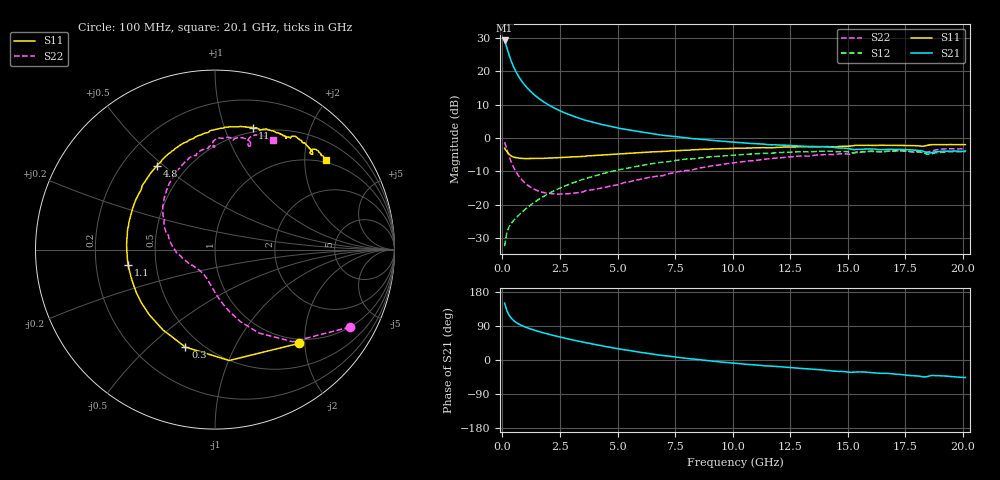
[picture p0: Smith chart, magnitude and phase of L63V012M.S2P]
!  Infineon Technologies AG
! BFR380L3 , PF131585-7, No.6, Th 09.10.01, soldered on pcb-board, measured with PP GSG850
!  Vce=3.0 V,  Ic=12.5 mA
! Common Emitter S-Parameters:  15. November 2001
#  GHz  S  MA  R  50
! f  S11  S21  S12  S22
! GHz  Mag  Ang  Mag  Ang  Mag  Ang  Mag  Ang
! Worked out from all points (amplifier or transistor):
!   201 points, 100 MHz to 20.1 GHz, reference 50 ohm
!   highest |S21| = 29.2 dB at 100 MHz (marker M1)
!   |S21| within 3 dB of that: start of sweep to 232.5 MHz
!   unconditionally stable (mu >= 1): 1.713 GHz to 4.436 GHz
!   at 3.4 GHz: K = 1.02, MAG = 8.2 dB, |S12| = -12.6 dB
!   at 10.1 GHz: K = 0.95, MSG = 1.9 dB, |S12| = -5.1 dB
!   at 20.1 GHz: K = 0.99, MSG = 0.1 dB, |S12| = -4.1 dB
!   S11 on the Smith chart (normalised r, x): 100 MHz: 0.91, -1.88; 300 MHz: 0.41, -0.66; 1.1 GHz: 0.34, -0.08; 4.8 GHz: 0.34, +0.47; 11 GHz: 0.45, +1.25; 20.1 GHz: 0.94, +2.54
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0.1  0.7017 -48.1  28.86 150.2  0.02392 66.7  0.8662 -29.9
0.2  0.623 -82.7  22.2 130.1  0.03847 56.7  0.6715 -49.9
0.3  0.5677 -106.9  17.2 117.8  0.04733 52.5  0.525 -62.3
0.4  0.5331 -123.0  13.8 109.6  0.05305 50.7  0.4254 -70.5
0.5  0.5156 -135.2  11.42 103.6  0.0585 51.1  0.3573 -76.6
0.6  0.5063 -143.8  9.716 99.2  0.06398 51.8  0.3093 -81.4
0.7  0.4997 -151.1  8.441 95.4  0.06904 52.9  0.2735 -85.4
0.8  0.4945 -156.9  7.462 92.2  0.07455 54.1  0.2463 -88.9
0.9  0.4923 -161.8  6.674 89.5  0.07998 55.2  0.2252 -92.0
1.1  0.4913 -169.9  5.527 84.6  0.09159 56.8  0.1963 -97.7
1.3  0.4901 -176.3  4.716 80.4  0.1032 58.0  0.1765 -102.7
1.5  0.4925 177.9  4.117 76.6  0.1152 58.7  0.1636 -107.3
2  0.5 166.7  3.14 68.2  0.146 59.0  0.1477 -118.4
2.6  0.5096 155.6  2.466 59.2  0.1833 57.8  0.1449 -130.6
3.5  0.5289 141.4  1.89 47.1  0.24 54.1  0.1552 -145.9
4.8  0.5676 124.8  1.464 32.1  0.3179 46.9  0.1929 -168.4
6.8  0.6259 103.5  1.121 13.2  0.4271 33.9  0.2697 163.6
10.1  0.7003 78.5  0.8618 -8.6  0.5553 12.3  0.4267 129.3
11  0.711 72.9  0.8213 -13.1  0.5806 6.6  0.4612 120.8
13.5  0.7387 60.4  0.7446 -24.3  0.625 -8.8  0.5465 100.4
16.8  0.7739 48.1  0.6752 -35.8  0.6312 -25.0  0.6358 78.6
20.1  0.7939 38.8  0.6362 -46.2  0.6239 -38.7  0.6909 62.0
